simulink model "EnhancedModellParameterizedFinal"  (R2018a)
settings: Solver=VariableStepAuto  StartTime=0.0  StopTime=Sim_time  RelTol=1e-3
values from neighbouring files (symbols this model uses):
  Amplitude_Signal = 5    [ParameterInitializationFileFinal.m]
  Anglog_Input_Max = 3    [ParameterInitializationFileFinal.m]    (also in Panda_BEVintage_VPE_S_Data_CodeGen_Model.m = 10; Panda_BEVintage_VPE_S_Data_Enhanced_Model.m = 10)
  Anglog_Input_Min = 0    [ParameterInitializationFileFinal.m]    (also in Panda_BEVintage_VPE_S_Data_CodeGen_Model.m = -10; Panda_BEVintage_VPE_S_Data_Enhanced_Model.m = -10)
  Bias_Signal = 0    [ParameterInitializationFileFinal.m]
  Bits = 12    [ParameterInitializationFileFinal.m]    (also in Panda_BEVintage_VPE_S_Data_CodeGen_Model.m = 16; Panda_BEVintage_VPE_S_Data_Enhanced_Model.m = 16)
  CutOff_Freq = Frequency_Signal*8    (= 4)    [ParameterInitializationFileFinal.m]
  Digital_Output = 3.3    [ParameterInitializationFileFinal.m]
  fclk = 10e4    (= 100000)    [ParameterInitializationFileFinal.m]
  fpwm = fclk/2^BitsPWM    (= 24.4140625)    [ParameterInitializationFileFinal.m]
  Frequency_Signal = 1/2    (= 0.5)    [ParameterInitializationFileFinal.m]
  Full_Scale_Reading = Anglog_Input_Max-Anglog_Input_Min    (= 3)    [ParameterInitializationFileFinal.m]    (also in Panda_BEVintage_VPE_S_Data_CodeGen_Model.m = 20; Panda_BEVintage_VPE_S_Data_Enhanced_Model.m = 20)
  Max_Signal = Amplitude_Signal+Bias_Signal    (= 5)    [ParameterInitializationFileFinal.m]
  Min_Signal = -Amplitude_Signal+Bias_Signal    (= -5)    [ParameterInitializationFileFinal.m]
  Sampling_Time = 0.01    [ParameterInitializationFileFinal.m]    (also in Panda_BEVintage_VPE_S_Data_CodeGen_Model.m = 0.0001; Panda_BEVintage_VPE_S_Data_Enhanced_Model.m = 0.0001)
libraries: dspfdesign x2, dsparch4 x1, pePwmGenerator x1

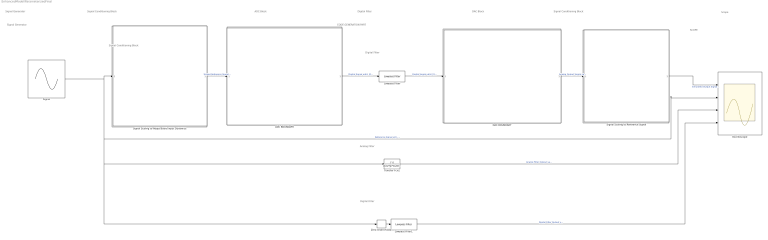
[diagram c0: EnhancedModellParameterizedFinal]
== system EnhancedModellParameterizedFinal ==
  note: Signal Conditioning Block
  note: Signal Conditioning Block
  note: CODE GENERATION PART
  note: SCOPE
  note: Analog Filter
  note: Signal Generator
  note: Digital Filter
  note: Digital Filter
  note: ADC Block
  note: Signal Generator
  note: Digital Filter
  note: DAC Block
  note: Signal Conditioning Block
  note: Scope
  ADC BOUNDARY : Subsystem
  DAC BOUNDARY : Subsystem
  Lowpass Filter : dspfdesign/Lowpass Filter  FilterType=IIR  DesignForMinimumOrder=off  FilterOrder=1  PassbandFrequency=Frequency_Signal*4  StopbandFrequency=1  PassbandRipple=1  StopbandAttenuation=80  InheritSampleRate=on  SampleRate=Frequency_Signal*5  SimulateUsing=Interpreted execution  roundingMode=Floor  coeffsDataTypeStr=fixdt(1,16)
  Lowpass Filter1 : dspfdesign/Lowpass Filter  FilterType=IIR  DesignForMinimumOrder=off  FilterOrder=1  PassbandFrequency=Frequency_Signal*4  StopbandFrequency=1  PassbandRipple=1  StopbandAttenuation=80  InheritSampleRate=on  SampleRate=Frequency_Signal/4  SimulateUsing=Interpreted execution  roundingMode=Floor  coeffsDataTypeStr=fixdt(1,16)
  Oscillioscope : Scope  NumInputPorts=4
  Signal : Sin  Amplitude=Amplitude_Signal  Bias=Bias_Signal  Frequency=2*pi*Frequency_Signal  SampleTime=0
  Signal Scaling to Adapt Board Input Dynamics : Subsystem
  Signal Scaling to Reference Signal : Subsystem
  Transfer Fcn2 : TransferFcn  Denominator=[1/(2*pi*CutOff_Freq) 1]
  Zero-Order Hold2 : ZeroOrderHold  SampleTime=Sampling_Time
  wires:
  Signal/1 -> Signal Scaling to Adapt Board Input Dynamics/1(Reference Signal u(t)), Oscillioscope/2, Zero-Order Hold2/1, Transfer Fcn2/1  "Reference Signal u(t) -5 To 5 [v]  1/2 [Hz]"
  Transfer Fcn2/1 -> Oscillioscope/3  "Analog Filter Output ya(t)"
  Signal Scaling to Adapt Board Input Dynamics/1(Scaled Reference Signal us(t)) -> ADC BOUNDARY/1(Scaled Reference Signal)  "Scaled Reference Signal us(t)"
  Signal Scaling to Reference Signal/1(Simulated Output Signal y(t) [-5 To 5] [V]) -> Oscillioscope/1  "Simulated Output Signal y(t) \t\t[-5 To 5] \t\t     [V]"
  ADC BOUNDARY/1("Digital Signal ud(z) [0-4095] 12 bits Sampling Time 0.01s ") -> Lowpass Filter/1  "Digital Signal ud(z) [0-4095] 12 bits  Sampling Time 0.01s"
  Lowpass Filter/1 -> DAC BOUNDARY/1("Digital Signal ud(z) [0-4095] 12 bits Sampling Time 0.01s  ")  "Digital Signal ud(z) [0-4095] 12 bits  Sampling Time 0.01s"
  DAC BOUNDARY/1(Analog Output Signal ya(t) [0-3.3] [V]) -> Signal Scaling to Reference Signal/1(Analog Output Signal ya(t) [0-3.3] [V])  "Analog Output Signal ya(t) [0-3.3] [V]"
  Lowpass Filter1/1 -> Oscillioscope/4  "Digital Filter Output yD(t)"
  Zero-Order Hold2/1 -> Lowpass Filter1/1

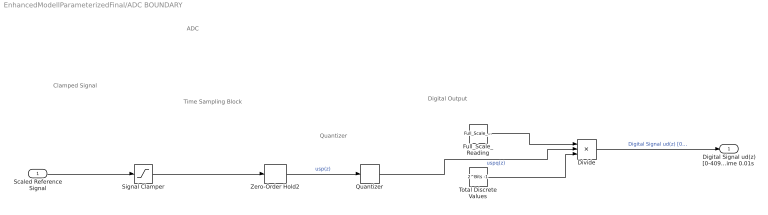
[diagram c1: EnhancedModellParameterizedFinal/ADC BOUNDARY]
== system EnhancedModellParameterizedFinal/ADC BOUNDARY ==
  note: Quantizer
  note: Time Sampling Block
  note: Digital Output
  note: Clamped Signal
  note: ADC
  Scaled Reference Signal : Inport
  Divide : Product  Inputs=/**
  Full_Scale_Reading : Constant  Value=Full_Scale_Reading
  Quantizer : Quantizer  QuantizationInterval=Full_Scale_Reading/(2^Bits-1 )
  Signal Clamper : Saturate  UpperLimit=Anglog_Input_Max  LowerLimit=0
  Total Discrete Values : Constant  Value=2^Bits -1
  Zero-Order Hold2 : ZeroOrderHold  SampleTime=Sampling_Time
  "Digital Signal ud(z) [0-4095] 12 bits Sampling Time 0.01s " : Outport
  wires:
  Signal Clamper/1 -> Zero-Order Hold2/1
  Scaled Reference Signal/1 -> Signal Clamper/1
  Full_Scale_Reading/1 -> Divide/1
  Total Discrete Values/1 -> Divide/3
  Quantizer/1 -> Divide/2  "uspq(z)"
  Divide/1 -> "Digital Signal ud(z) [0-4095] 12 bits Sampling Time 0.01s "/1  "Digital Signal ud(z) [0-4095] 12 bits  Sampling Time 0.01s"
  Zero-Order Hold2/1 -> Quantizer/1  "usp(z)"

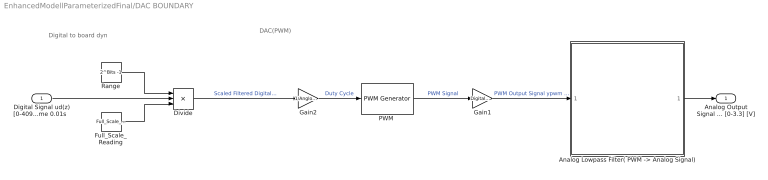
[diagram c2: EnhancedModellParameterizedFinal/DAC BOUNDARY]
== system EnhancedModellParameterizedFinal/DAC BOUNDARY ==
  note: DAC(PWM)
  note: Digital to board dyn
  "Digital Signal ud(z) [0-4095] 12 bits Sampling Time 0.01s  " : Inport
  "Analog Lowpass Filter( PWM -> Analog Signal)" : Subsystem
  Divide : Product  Inputs=/**
  Full_Scale_Reading : Constant  Value=Full_Scale_Reading
  Gain1 : Gain  Gain=Digital_Output
  Gain2 : Gain  Gain=1/Anglog_Input_Max
  "PWM " : pePwmGenerator/PWM Generator  CarrCount=Up  Tper=1/fpwm  Ts=1/fclk
  Range : Constant  Value=2^Bits -1
  Analog Output Signal ya(t) [0-3.3] [V] : Outport
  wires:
  Gain2/1 -> "PWM "/1  "Duty Cycle"
  "PWM "/1 -> Gain1/1  "PWM Signal"
  Gain1/1 -> "Analog Lowpass Filter( PWM -> Analog Signal)"/1("PWM  Signal ")  "PWM Output Signal ypwm \t\t[0-1]"
  Range/1 -> Divide/1
  Full_Scale_Reading/1 -> Divide/3
  "Digital Signal ud(z) [0-4095] 12 bits Sampling Time 0.01s  "/1 -> Divide/2
  Divide/1 -> Gain2/1  "Scaled Filtered Digital Output yds(z) \t\t\t[0-3] \t\t\t [V]"
  "Analog Lowpass Filter( PWM -> Analog Signal)"/1(ya(t)) -> Analog Output Signal ya(t) [0-3.3] [V]/1

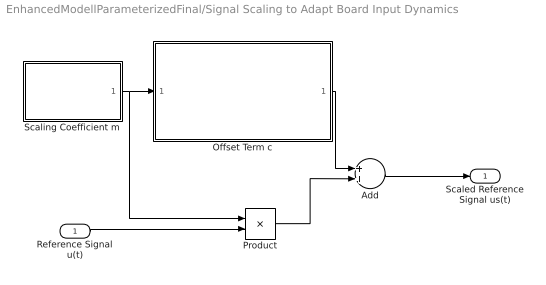
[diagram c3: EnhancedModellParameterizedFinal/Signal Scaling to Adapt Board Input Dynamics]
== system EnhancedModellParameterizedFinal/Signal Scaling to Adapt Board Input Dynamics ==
  Reference Signal u(t) : Inport
  Add : Sum
  Offset Term c : Subsystem
  Product : Product
  Scaling Coefficient m : Subsystem
  Scaled Reference Signal us(t) : Outport
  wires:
  Scaling Coefficient m/1(Scaling Coefficient m) -> Product/1, Offset Term c/1(Scaling Coefficent m)
  Reference Signal u(t)/1 -> Product/2
  Product/1 -> Add/2
  Offset Term c/1("Offset Term c ") -> Add/1
  Add/1 -> Scaled Reference Signal us(t)/1

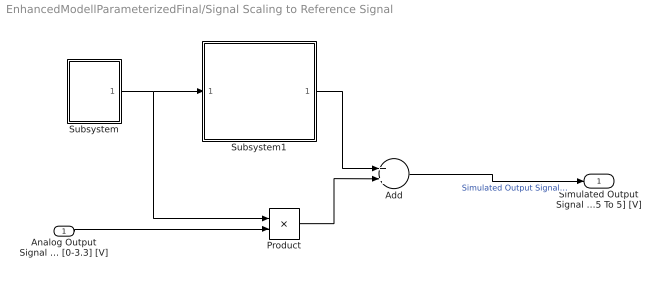
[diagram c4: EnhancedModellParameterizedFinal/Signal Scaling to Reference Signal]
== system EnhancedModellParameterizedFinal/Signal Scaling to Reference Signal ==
  Analog Output Signal ya(t) [0-3.3] [V] : Inport
  Add : Sum
  Product : Product
  Subsystem : Subsystem
  Subsystem1 : Subsystem
  Simulated Output Signal y(t) [-5 To 5] [V] : Outport
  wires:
  Product/1 -> Add/2
  Add/1 -> Simulated Output Signal y(t) [-5 To 5] [V]/1  "Simulated Output Signal y(t) \t\t[-5 To 5] \t\t     [V]"
  Subsystem/1("Gradient ") -> Product/1, Subsystem1/1("Gradient ")
  Subsystem1/1("Offset ") -> Add/1
  Analog Output Signal ya(t) [0-3.3] [V]/1 -> Product/2

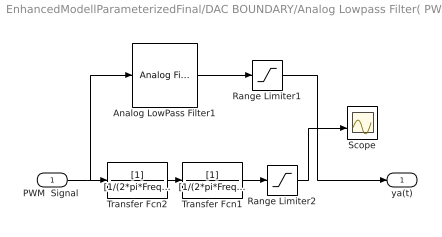
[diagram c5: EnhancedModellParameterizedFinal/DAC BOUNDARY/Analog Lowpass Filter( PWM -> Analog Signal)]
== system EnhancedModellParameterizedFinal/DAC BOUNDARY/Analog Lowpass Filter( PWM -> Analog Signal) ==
  "PWM  Signal " : Inport
  Analog LowPass Filter1 : dsparch4/Analog Filter Design  method=Butterworth  filttype=Lowpass  N=2  Wlo=2*pi*Frequency_Signal*4  Whi=80  Rp=2  Rs=40
  Range Limiter1 : Saturate  UpperLimit=Digital_Output  LowerLimit=0
  Range Limiter2 : Saturate  Commented=on  UpperLimit=Digital_Output  LowerLimit=0
  Scope : Scope  NumInputPorts=2
  Transfer Fcn1 : TransferFcn  Commented=on  Denominator=[1/(2*pi*Frequency_Signal*5) 1]
  Transfer Fcn2 : TransferFcn  Commented=on  Denominator=[1/(2*pi*Frequency_Signal*5) 1]
  ya(t) : Outport
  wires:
  Range Limiter2/1 -> Scope/2
  "PWM  Signal "/1 -> Analog LowPass Filter1/1, Transfer Fcn2/1
  Analog LowPass Filter1/1 -> Range Limiter1/1
  Range Limiter1/1 -> ya(t)/1
  Transfer Fcn2/1 -> Transfer Fcn1/1
  Transfer Fcn1/1 -> Range Limiter2/1

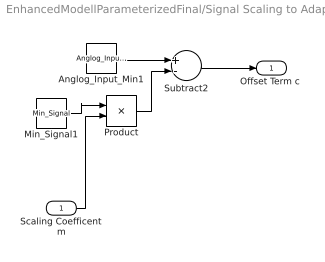
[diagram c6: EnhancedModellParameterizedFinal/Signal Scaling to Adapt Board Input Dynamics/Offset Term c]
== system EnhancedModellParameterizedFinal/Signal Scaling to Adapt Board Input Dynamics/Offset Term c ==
  Scaling Coefficent m : Inport
  Anglog_Input_Min1 : Constant  Value=Anglog_Input_Min
  Min_Signal1 : Constant  Value=Min_Signal
  Product : Product
  Subtract2 : Sum  Inputs=+-
  "Offset Term c " : Outport
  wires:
  Min_Signal1/1 -> Product/1
  Scaling Coefficent m/1 -> Product/2
  Product/1 -> Subtract2/2
  Subtract2/1 -> "Offset Term c "/1
  Anglog_Input_Min1/1 -> Subtract2/1

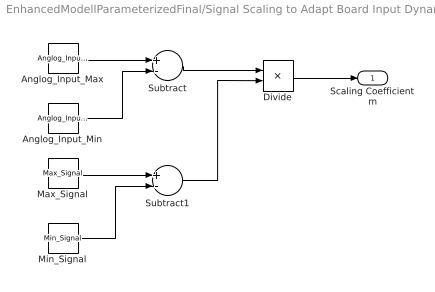
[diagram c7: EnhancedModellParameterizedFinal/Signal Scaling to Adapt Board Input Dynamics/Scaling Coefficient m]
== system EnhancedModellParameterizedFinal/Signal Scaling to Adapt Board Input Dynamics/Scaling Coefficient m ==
  Anglog_Input_Max : Constant  Value=Anglog_Input_Max
  Anglog_Input_Min : Constant  Value=Anglog_Input_Min
  Divide : Product  Inputs=*/
  Max_Signal : Constant  Value=Max_Signal
  Min_Signal : Constant  Value=Min_Signal
  Subtract : Sum  Inputs=+-
  Subtract1 : Sum  Inputs=+-
  Scaling Coefficient m : Outport
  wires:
  Divide/1 -> Scaling Coefficient m/1
  Subtract1/1 -> Divide/2
  Subtract/1 -> Divide/1
  Anglog_Input_Min/1 -> Subtract/2
  Min_Signal/1 -> Subtract1/2
  Max_Signal/1 -> Subtract1/1
  Anglog_Input_Max/1 -> Subtract/1

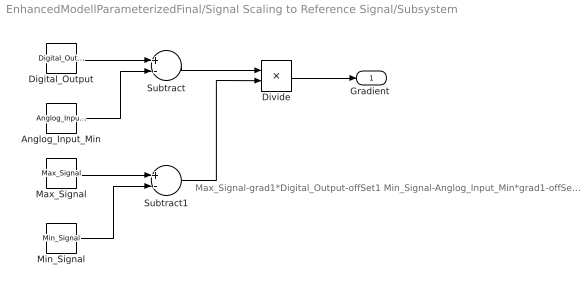
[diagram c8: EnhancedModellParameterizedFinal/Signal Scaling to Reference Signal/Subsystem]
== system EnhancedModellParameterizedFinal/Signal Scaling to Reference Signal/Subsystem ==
  note: Max_Signal-grad1*Digital_Output-offSet1 Min_Signal-Anglog_Input_Min*grad1-offSet1
  Anglog_Input_Min : Constant  Value=Anglog_Input_Min
  Digital_Output : Constant  Value=Digital_Output
  Divide : Product  Inputs=/*
  Max_Signal : Constant  Value=Max_Signal
  Min_Signal : Constant  Value=Min_Signal
  Subtract : Sum  Inputs=+-
  Subtract1 : Sum  Inputs=+-
  "Gradient " : Outport
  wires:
  Divide/1 -> "Gradient "/1
  Subtract1/1 -> Divide/2
  Subtract/1 -> Divide/1
  Anglog_Input_Min/1 -> Subtract/2
  Min_Signal/1 -> Subtract1/2
  Max_Signal/1 -> Subtract1/1
  Digital_Output/1 -> Subtract/1

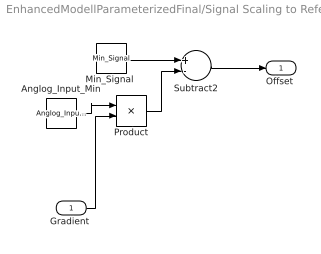
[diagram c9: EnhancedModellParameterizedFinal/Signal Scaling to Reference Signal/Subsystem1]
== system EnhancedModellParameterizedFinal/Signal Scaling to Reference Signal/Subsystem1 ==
  "Gradient " : Inport
  Anglog_Input_Min : Constant  Value=Anglog_Input_Min
  "Min_Signal " : Constant  Value=Min_Signal
  Product : Product
  Subtract2 : Sum  Inputs=+-
  "Offset " : Outport
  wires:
  Anglog_Input_Min/1 -> Product/1
  "Gradient "/1 -> Product/2
  Product/1 -> Subtract2/2
  Subtract2/1 -> "Offset "/1
  "Min_Signal "/1 -> Subtract2/1
